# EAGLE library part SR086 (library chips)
Adjustable Off-Line Inductorless Switching Regulator
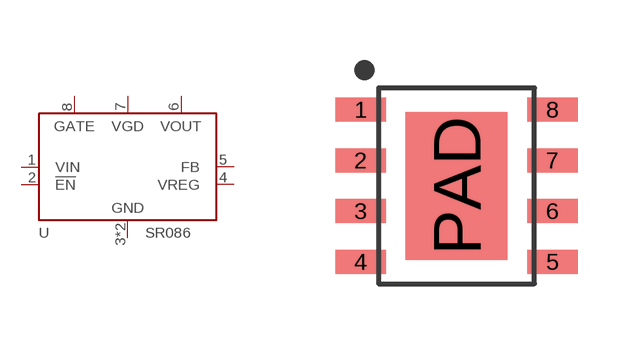
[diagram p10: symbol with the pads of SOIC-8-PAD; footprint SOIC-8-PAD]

Designator prefix U

## SR086SG-G (MOUSER: 689-SR086SG-G)  [SOIC-8-PAD]
1  VIN
2  !EN
3  GND
4  VREG
5  FB
6  VOUT
7  VGD
8  GATE
PAD  GND

## Footprint SOIC-8-PAD (pad centres in mm)
smd 1.27 x 0.6: 1 -2.4,1.905; 2 -2.4,0.635; 3 -2.4,-0.635; 4 -2.4,-1.905; 5 2.4,-1.905; 6 2.4,-0.635; 7 2.4,0.635; 8 2.4,1.905
smd 2.55 x 3.7: PAD 0,0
